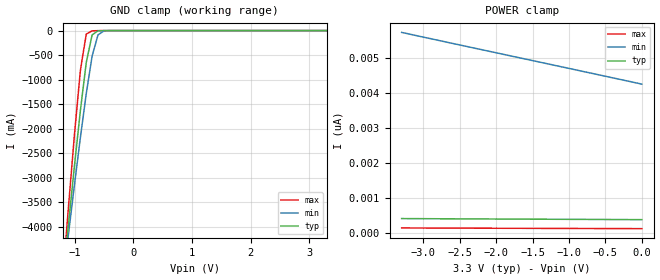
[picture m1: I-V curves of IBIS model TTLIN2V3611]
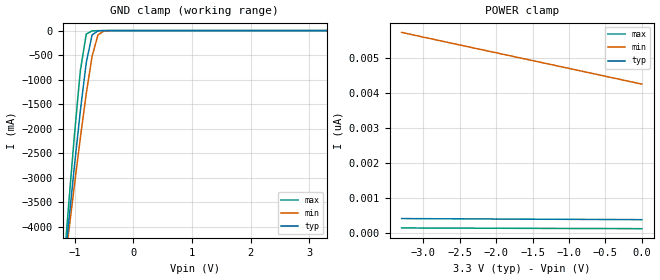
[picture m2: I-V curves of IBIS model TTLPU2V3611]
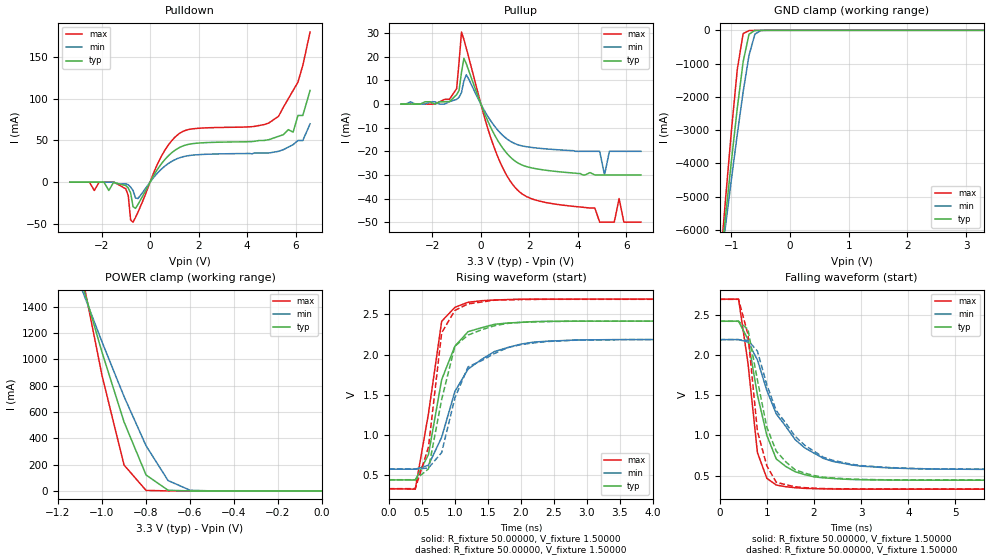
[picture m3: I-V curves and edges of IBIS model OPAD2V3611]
| IBIS file 36110bb.ibs created by s2ibis2 version 1.2
| North Carolina State University Electronics Research Laboratory  1995
[IBIS ver]   2.1
[File name]   36110bb.ibs
[File Rev]   1.0
[Date]   Friday, April 4, 2003
[Source]   IDT
[Notes]   1. Temp typ=25C, min=-40C, max=85C
   2. IDT C11_5_3.3V_SAC_2M process
   3. Ramp rates based on 50 ohm load
[Disclaimer]
READ THESE TERMS AND CONDITIONS CAREFULLY BEFORE USING THIS IBIS MODEL.  BY
USING THIS IBIS MODEL, YOU ARE ACCEPTING AND AGREEING TO THESE TERMS AND
CONDITIONS OF USE.
Integrated Device Technology, Inc. ("IDT") hereby grants the user of this
IBIS model ("User") a non-exclusive, nontransferable license to use this
IBIS model under the following terms: The User is granted this license only
to use the IBIS model for demonstration purposes only and is not granted
rights to sell, copy (except as needed to run the IBIS model), rent, lease
or sub-license (except for demonstration) the IBIS model in whole or in
part, or in modified form to anyone. The User may modify the IBIS model to
suit its specific applications, but  rights to derivative works and such
modifications shall belong to IDT.
THIS IBIS MODEL IS PROVIDED ON AN AS IS" BASIS AND IDT  MAKES ABSOLUTELY NO
WARRANTY WITH RESPECT TO THE INFORMATION CONTAINED HEREIN.  IDT DISCLAIMS
AND USER WAIVES ALL WARRANTIES, EXPRESS AND IMPLIED, INCLUDING WARRANTIES OF
MERCHANTABILITY AND FITNESS FOR A PARTICULAR PURPOSE.  THE ENTIRE RISK AS TO
QUALITY AND PERFORMANCE IS WITH THE USER  ACCORDINGLY, IN NO EVENT SHALL IDT
BE LIABLE FOR ANY DIRECT OR INDIRECT DAMAGES, WHETHER IN CONTRACT OR TORT,
INCLUDING ANY LOST PROFITS OR OTHER INCIDENTAL, CONSEQUENTIAL, EXEMPLARY, OR
PUNITIVE DAMAGES ARISING OUT OF THE USE OR APPLICATION OF THE  IBIS MODEL,
WHETHER OR NOT IDT HAD NOTICE OF SUCH DAMAGES.
IDT reserves the right to make changes without notice to any product herein
to improve reliability, function, or design. IDT does not convey any license
under patent rights or any other intellectual property rights, including
those of third parties. IDT is not obligated to provide maintenance or
support for the licensed IBIS model.
This model is for the 3.3v High-Density Supersync II 36-Bit FIFO
[Copyright]
Copyright 2002, Integrated Device Technology, Inc. All rights reserved.
|   Component 36110BB
[Component]   36110BB
[Manufacturer]   Integrated Device Technology Inc.
[Package]
|Following package parameters are for 144 lead PBGA package
| variable   typ   min   max
R_pkg   0.18000   0.10500   0.20900
L_pkg   8.10000nH   7.30000nH   9.90000nH
C_pkg   0.53000pF   0.46000pF   0.60000pF
[Pin]  signal_name   model_name   R_pin   L_pin   C_pin
1A   /ASYW   TTLIN2V3611
1B   /SEN   TTLIN2V3611
1C   D35   TTLIN2V3611
1D   D32   TTLIN2V3611
1E   D29   TTLIN2V3611
1F   D26   TTLIN2V3611
1G   D21   TTLIN2V3611
1H   D18   TTLIN2V3611
1J   D15   TTLIN2V3611
1K   D12   TTLIN2V3611
1L   D10   TTLIN2V3611
1M   D9   TTLIN2V3611
2A   /WEN   TTLIN2V3611
2B   IW   TTLIN2V3611
2C   D34   TTLIN2V3611
2D   D31   TTLIN2V3611
2E   D28   TTLIN2V3611
2F   D25   TTLIN2V3611
2G   D22   TTLIN2V3611
2H   D19   TTLIN2V3611
2J   D16   TTLIN2V3611
2K   D13   TTLIN2V3611
2L   D11   TTLIN2V3611
2M   D8   TTLIN2V3611
3A   RCLK   TTLIN2V3611
3B   /PRS   TTLIN2V3611
3C   D33   TTLIN2V3611
3D   D30   TTLIN2V3611
3E   D27   TTLIN2V3611
3F   D24   TTLIN2V3611
3G   D23   TTLIN2V3611
3H   D20   TTLIN2V3611
3J   D17   TTLIN2V3611
3K   D14   TTLIN2V3611
3L   D6   TTLIN2V3611
3M   D7   TTLIN2V3611
4A   /PAF   OPAD2V3611
4B   /LD   TTLIN2V3611
4C   FWFT/SI   TTLIN2V3611
4D   VCC   POWER
4E   VCC   POWER
4F   VCC   POWER
4G   VCC   POWER
4H   VCC   POWER
4J   VCC   POWER
4K   D3   TTLIN2V3611
4L   D4   TTLIN2V3611
4M   D5   TTLIN2V3611
5A   /FF-/IR   OPAD2V3611
5B   /MRS   TTLIN2V3611
5C   OW   TTLIN2V3611
5D   VCC   POWER
5E   GND   GND
5F   GND   GND
5G   GND   GND
5H   GND   GND
5J   VCC   POWER
5K   D0   TTLIN2V3611
5L   D1   TTLIN2V3611
5M   D2   TTLIN2V3611
6A   /HF   OPAD2V3611
6B   FS0   TTLIN2V3611
6C   VCC   POWER
6D   GND   GND
6E   GND   GND
6F   GND   GND
6G   GND   GND
6H   GND   GND
6J   GND   GND
6K   VCC   POWER
6L   TMS   TTLPU2V3611
6M   /TRST   TTLPU2V3611
7A   BM   TTLIN2V3611
7B   FS1   TTLIN2V3611
7C   VCC   POWER
7D   GND   GND
7E   GND   GND
7F   GND   GND
7G   GND   GND
7H   GND   GND
7J   GND   GND
7K   VCC   POWER
7L   TCK   TTLIN2V3611
7M   TDI   TTLPU2V3611
8A   /EF   OPAD2V3611
8B   /ASYR   TTLIN2V3611
8C   /BE   TTLIN2V3611
8D   VCC   POWER
8E   GND   GND
8F   GND   GND
8G   GND   GND
8H   GND   GND
8J   VCC   POWER
8K   TDO   FLOPAD2V3611
8L   Q0   OPAD2V3611
8M   Q1   OPAD2V3611
9A   RCLK   TTLIN2V3611
9B   IP   TTLIN2V3611
9C   /PAE   OPAD2V3611
9D   VCC   POWER
9E   VCC   POWER
9F   VCC   POWER
9G   VCC   POWER
9H   VCC   POWER
9J   VCC   POWER
9K   Q2   OPAD2V3611
9L   Q3   OPAD2V3611
9M   Q4   OPAD2V3611
10A   /REN   TTLIN2V3611
10B   PFM   TTLIN2V3611
10C   RM   TTLIN2V3611
10D   Q29   OPAD2V3611
10E   Q26   OPAD2V3611
10F   Q23   OPAD2V3611
10G   Q22   OPAD2V3611
10H   Q19   OPAD2V3611
10J   Q16   OPAD2V3611
10K   Q13   OPAD2V3611
10L   Q5   OPAD2V3611
10M   Q6   OPAD2V3611
11A   /OE   TTLIN2V3611
11B   /RT   TTLIN2V3611
11C   Q32   OPAD2V3611
11D   Q30   OPAD2V3611
11E   Q27   OPAD2V3611
11F   Q24   OPAD2V3611
11G   Q21   OPAD2V3611
11H   Q18   OPAD2V3611
11J   Q15   OPAD2V3611
11K   Q12   OPAD2V3611
11L   Q10   OPAD2V3611
11M   Q7   OPAD2V3611
12A   Q35   OPAD2V3611
12B   Q34   OPAD2V3611
12C   Q33   OPAD2V3611
12D   Q31   OPAD2V3611
12E   Q28   OPAD2V3611
12F   Q25   OPAD2V3611
12G   Q20   OPAD2V3611
12H   Q17   OPAD2V3611
12J   Q14   OPAD2V3611
12K   Q11   OPAD2V3611
12L   Q9   OPAD2V3611
12M   Q8   OPAD2V3611
| Models and submodels in the file (4): TTLIN2V3611 (Input), TTLPU2V3611 (Input), OPAD2V3611 (3-state), FLOPAD2V3611 (3-state)
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| in   in   dummy_model
| oe   oe   dummy_model
| in1  in1   dummy_model
| oe1  oe1   dummy_model
|   Model TTLIN2V3611
[Model]   TTLIN2V3611
Model_type   Input
Polarity   Non-Inverting
Vinl =  0.80000V
Vinh =  2.00000V
C_comp   10.00000pF   10.00000pF   10.00000pF
[Temperature Range]   25.00000   85.00000   -40.00000
[Voltage Range]   3.30000V   3.15000V   3.45000V
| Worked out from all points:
|   GND clamp passes 1 mA (typ) near -0.51 V on its own axis
[GND_clamp]
| voltage   I(typ)   I(min)   I(max)
-3.3V     -31.62A    -27.14A    -38.3A
-1.2V     -5.12A     -5.123A    -5.052A
-1.1V     -3.918A    -4.12A     -3.553A
-1V       -2.746A    -3.136A    -2.109A
-900mV    -1.631A    -2.183A    -811.7mA
-800mV    -652.4mA   -1.286A    -71.19mA
-700mV    -87.47mA   -520.5mA   -5.646mA
-600mV    -5.364mA   -87.77mA   -1.458mA
-500mV    -302uA     -8.09mA    -219uA
3.3V      373pA      4.31nA     115.1pA
[POWER_clamp]
| voltage   I(typ)   I(min)   I(max)
-3.3V     403.8pA    5.719nA    136.4pA
-2.6V     396.7pA    5.404nA    131.5pA
-1.3V     385pA      4.825nA    123.6pA
0V        373pA      4.243nA    116pA
|   Model TTLPU2V3611
[Model]   TTLPU2V3611
Model_type   Input
Polarity   Non-Inverting
Vinl =  0.80000V
Vinh =  2.00000V
C_comp   10.00000pF   10.00000pF   10.00000pF
[Temperature Range]   25.00000   85.00000   -40.00000
[Voltage Range]   3.30000V   3.15000V   3.45000V
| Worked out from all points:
|   GND clamp passes 1 mA (typ) near -0.51 V on its own axis
[GND_clamp]
| voltage   I(typ)   I(min)   I(max)
-3.3V     -31.62A    -27.14A    -38.3A
-1.2V     -5.12A     -5.123A    -5.052A
-1.1V     -3.918A    -4.12A     -3.553A
-1V       -2.746A    -3.136A    -2.109A
-900mV    -1.631A    -2.183A    -811.7mA
-800mV    -652.4mA   -1.286A    -71.2mA
-700mV    -87.48mA   -520.5mA   -5.659mA
-600mV    -5.37mA    -87.77mA   -1.473mA
-500mV    -314.2uA   -8.094mA   -239.3uA
3.3V      373pA      4.31nA     115.1pA
[POWER_clamp]
| voltage   I(typ)   I(min)   I(max)
-3.3V     403.8pA    5.719nA    136.4pA
-2.6V     396.7pA    5.404nA    131.5pA
-1.3V     385pA      4.825nA    123.6pA
0V        373pA      4.243nA    116pA
|   Model OPAD2V3611
[Model]   OPAD2V3611
Model_type   3-state
Polarity   Non-Inverting
Enable   Active-High
Vmeas =  1.50000V
C_comp   10.00000pF   10.00000pF   10.00000pF
[Temperature Range]   25.00000   85.00000   -40.00000
[Voltage Range]   3.30000V   3.15000V   3.45000V
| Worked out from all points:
|   slope of the pulldown table from 0 to 0.495 V, typ, clamps not added: 21.5 ohm
|   slope of the pullup table from 0 to 0.495 V, typ, clamps not added: 42.4 ohm
|   GND clamp passes 1 mA (typ) near -0.52 V on its own axis
|   POWER clamp passes 1 mA (typ) near -0.62 V on its own axis
|   rising waveform, R_fixture 50.00000, V_fixture 1.50000: 20-80 % time 343ps typ, 520ps min, 265ps max; typ from 0.444 V to 2.42 V
|   rising waveform, R_fixture 50.00000, V_fixture 1.50000: 20-80 % time 315ps typ, 412ps min, 210ps max; typ from 0.447 V to 2.42 V
|   falling waveform, R_fixture 50.00000, V_fixture 1.50000: 20-80 % time 461ps typ, 858ps min, 278ps max; typ from 2.42 V to 0.444 V
|   falling waveform, R_fixture 50.00000, V_fixture 1.50000: 20-80 % time 482ps typ, 874ps min, 309ps max; typ from 2.42 V to 0.447 V
[Pulldown]
| voltage   I(typ)   I(min)   I(max)
-3.3V     0A         0A         0A
-1V       -4mA       -2mA       -8mA
-800mV    -13.1mA    -6mA       -45.44mA
-700mV    -29.4mA    -10mA      -47.99mA
-500mV    -26.74mA   -19.63mA   -36.09mA
400mV     19.36mA    13.74mA    27.32mA
1.2V      41.38mA    29.07mA    58.2mA
5.3V      55mA       37mA       79mA
5.9V      60mA       45mA       110mA
6.1V      80mA       50mA       120mA
6.3V      80mA       50mA       140mA
6.6V      110mA      70mA       180mA
[Pullup]
| voltage   I(typ)   I(min)   I(max)
-3.3V     0A         0A         0A
-1.3V     1mA        1mA        2mA
-1V       4mA        2mA        6.5mA
-800mV    13.4mA     4.9mA      30.49mA
-600mV    17.05mA    12.41mA    23.59mA
500mV     -11.77mA   -8.469mA   -17mA
1.5V      -24.75mA   -17.12mA   -36.28mA
4.9V      -30mA      -20mA      -50mA
5.1V      -30mA      -30mA      -50mA
5.7V      -30mA      -20mA      -40mA
5.9V      -30mA      -20mA      -50mA
6.6V      -30mA      -20mA      -50mA
[GND_clamp]
| voltage   I(typ)   I(min)   I(max)
-3.3V     -44.86A    -38.5A     -54.32A
-1.2V     -7.292A    -7.294A    -7.196A
-1.1V     -5.587A    -5.872A    -5.069A
-1V       -3.924A    -4.477A    -3.02A
-900mV    -2.338A    -3.123A    -1.172A
-800mV    -940.2mA   -1.846A    -98.36mA
-700mV    -115.7mA   -749mA     -8.05mA
-600mV    -4.278mA   -114.8mA   -2.238mA
-500mV    -295.2uA   -5.816mA   -325.4uA
3.3V      607.7pA    5.602nA    92.71pA
[POWER_clamp]
| voltage   I(typ)   I(min)   I(max)
-3.3V     15.46A     11.9A      22.55A
-1.1V     1.627A     1.567A     1.714A
-1V       1.053A     1.131A     875.2mA
-900mV    523.9mA    716.9mA    196.8mA
-800mV    121.2mA    343.1mA    4.086mA
-700mV    5.031mA    78.95mA    112.4uA
-600mV    111.5uA    5.081mA    8.814uA
0V        607.7pA    2.814nA    110.2pA
[Ramp]
| variable   typ   min   max
dV/dt_r   0.80040/0.49852n   0.55518/0.74186n   1.11420/0.33285n
dV/dt_f   1.24980/0.73875n   0.95160/1.28926n   1.51836/0.39958n
R_load = 50.00000
[Rising Waveform]
R_fixture = 50.00000
V_fixture = 1.50000
V_fixture_min = 1.50000
V_fixture_max = 1.50000
| time   V(typ)   V(min)   V(max)
0s        444.1mV    577.5mV    332.7mV
400ps     443.2mV    577.5mV    329.4mV
600ps     759mV      626.9mV    1.268V
800ps     1.69V      974.8mV    2.415V
1ns       2.105V     1.542V     2.588V
1.2ns     2.286V     1.821V     2.651V
1.6ns     2.377V     2.039V     2.679V
2ns       2.402V     2.131V     2.689V
2.4ns     2.414V     2.167V     2.69V
10ns      2.417V     2.189V     2.691V
[Rising Waveform]
R_fixture = 50.00000
V_fixture = 1.50000
V_fixture_min = 1.50000
V_fixture_max = 1.50000
R_dut = 0.18000
L_dut = 8.10000nH
C_dut = 0.53000pF
| time   V(typ)   V(min)   V(max)
0s        446.6mV    579.4mV    335.9mV
400ps     446.6mV    579.4mV    335.6mV
600ps     581mV      592.2mV    852.1mV
800ps     1.444V     784.2mV    2.272V
1ns       2.105V     1.463V     2.551V
1.2ns     2.244V     1.849V     2.631V
1.6ns     2.36V      2.014V     2.678V
1.8ns     2.389V     2.088V     2.682V
2.4ns     2.412V     2.164V     2.688V
10ns      2.416V     2.188V     2.688V
[Falling Waveform]
R_fixture = 50.00000
V_fixture = 1.50000
V_fixture_min = 1.50000
V_fixture_max = 1.50000
| time   V(typ)   V(min)   V(max)
0s        2.417V     2.189V     2.691V
400ps     2.417V     2.189V     2.692V
600ps     2.192V     2.159V     1.896V
800ps     1.502V     1.937V     786.7mV
1ns       1V         1.557V     467.2mV
1.2ns     707.2mV    1.267V     383.9mV
1.8ns     513.6mV    846.8mV    342.6mV
2.2ns     473.3mV    714.4mV    336.7mV
2.8ns     452.6mV    633mV      333.3mV
10ns      444.1mV    577.6mV    332.7mV
[Falling Waveform]
R_fixture = 50.00000
V_fixture = 1.50000
V_fixture_min = 1.50000
V_fixture_max = 1.50000
R_dut = 0.18000
L_dut = 8.10000nH
C_dut = 0.53000pF
| time   V(typ)   V(min)   V(max)
0s        2.416V     2.188V     2.688V
400ps     2.416V     2.188V     2.688V
600ps     2.316V     2.179V     2.251V
800ps     1.688V     2.046V     1.053V
1ns       1.101V     1.627V     621.5mV
1.2ns     804.3mV    1.307V     418.5mV
1.8ns     531.8mV    879.3mV    351.2mV
2.2ns     481.7mV    728.8mV    340.3mV
3ns       454mV      624.9mV    336.2mV
10ns      446.6mV    579.4mV    335.9mV
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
